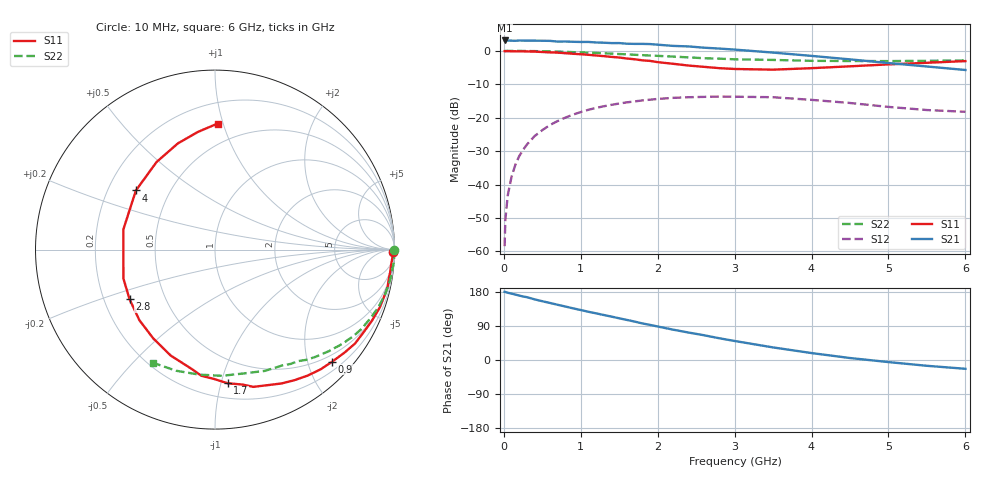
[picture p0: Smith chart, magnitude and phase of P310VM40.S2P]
! SIEMENS Small Signal Semiconductors
! BFP181
! Si NPN RF Bipolar Junction Transistor in SOT143
! VCE = 10 V  IC = 0.4 mA
! Common Emitter S-Parameters:  March  1996
# GHz  S  MA  R  50
!  f  S11  S21  S12  S22
! GHz  MAG  ANG  MAG  ANG  MAG  ANG  MAG  ANG
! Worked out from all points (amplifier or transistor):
!   36 points, 10 MHz to 6 GHz, reference 50 ohm
!   highest |S21| = 3.1 dB at 10 MHz (marker M1)
!   |S21| within 3 dB of that: start of sweep to 3.148 GHz
!   unconditionally stable (mu >= 1): 3.905 GHz to end of sweep
!   at 250 MHz: K = 0.09, MSG = 16.3 dB, |S12| = -29.6 dB
!   at 1.4 GHz: K = 0.42, MSG = 9.2 dB, |S12| = -16.1 dB
!   at 6 GHz: K = 1.47, MAG = 2.2 dB, |S12| = -18.2 dB
!   S11 on the Smith chart (normalised r, x): 10 MHz: open; 900 MHz: 0.36, -2.45; 1.7 GHz: 0.31, -1.05; 2.8 GHz: 0.31, -0.25; 4 GHz: 0.32, +0.30; 6 GHz: 0.35, +0.96
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0.01  0.9894 -0.7  1.429 179.8  0.0012 88.6  0.9988 -0.2
0.02  0.9857 -1.1  1.419 179.6  0.003 87.7  0.9975 -0.4
0.05  0.9904 -2.2  1.426 177.5  0.0068 90.2  0.9976 -1.3
0.1  0.9847 -5.0  1.418 175.2  0.0131 85.3  0.9995 -2.5
0.15  0.9839 -7.4  1.412 172.7  0.0198 84.7  0.9973 -3.6
0.2  0.9821 -9.7  1.427 170.0  0.0267 82.9  0.9969 -4.9
0.3  0.9795 -14.6  1.418 165.8  0.0397 79.2  0.9934 -7.3
0.5  0.9601 -24.4  1.414 155.1  0.0652 71.7  0.9855 -12.2
0.9  0.9034 -43.7  1.365 136.3  0.1113 57.8  0.9557 -21.5
1.1  0.8712 -53.7  1.358 127.2  0.1314 51.4  0.9378 -25.8
1.5  0.794 -74.4  1.306 110.0  0.163 38.9  0.8951 -34.2
1.7  0.7481 -84.6  1.27 101.4  0.1754 33.1  0.8726 -38.0
1.9  0.707 -96.2  1.262 92.7  0.186 27.5  0.851 -41.6
2.2  0.6398 -112.7  1.185 80.1  0.198 19.8  0.8199 -46.7
2.4  0.6026 -124.8  1.164 72.5  0.2024 14.5  0.7981 -50.3
2.8  0.5506 -149.8  1.081 57.4  0.207 5.5  0.7636 -56.5
3  0.5352 -162.4  1.043 50.2  0.2061 1.0  0.7469 -59.7
3.5  0.5229 167.7  0.941 33.2  0.2024 -8.8  0.7308 -67.6
4  0.5502 143.2  0.84 18.3  0.1848 -16.6  0.7085 -76.8
4.5  0.5867 123.7  0.745 5.2  0.166 -22.6  0.7043 -86.9
5.5  0.6624 98.3  0.583 -15.3  0.1302 -22.6  0.7088 -107.8
6  0.7025 88.8  0.517 -23.2  0.1226 -18.6  0.7193 -118.8
